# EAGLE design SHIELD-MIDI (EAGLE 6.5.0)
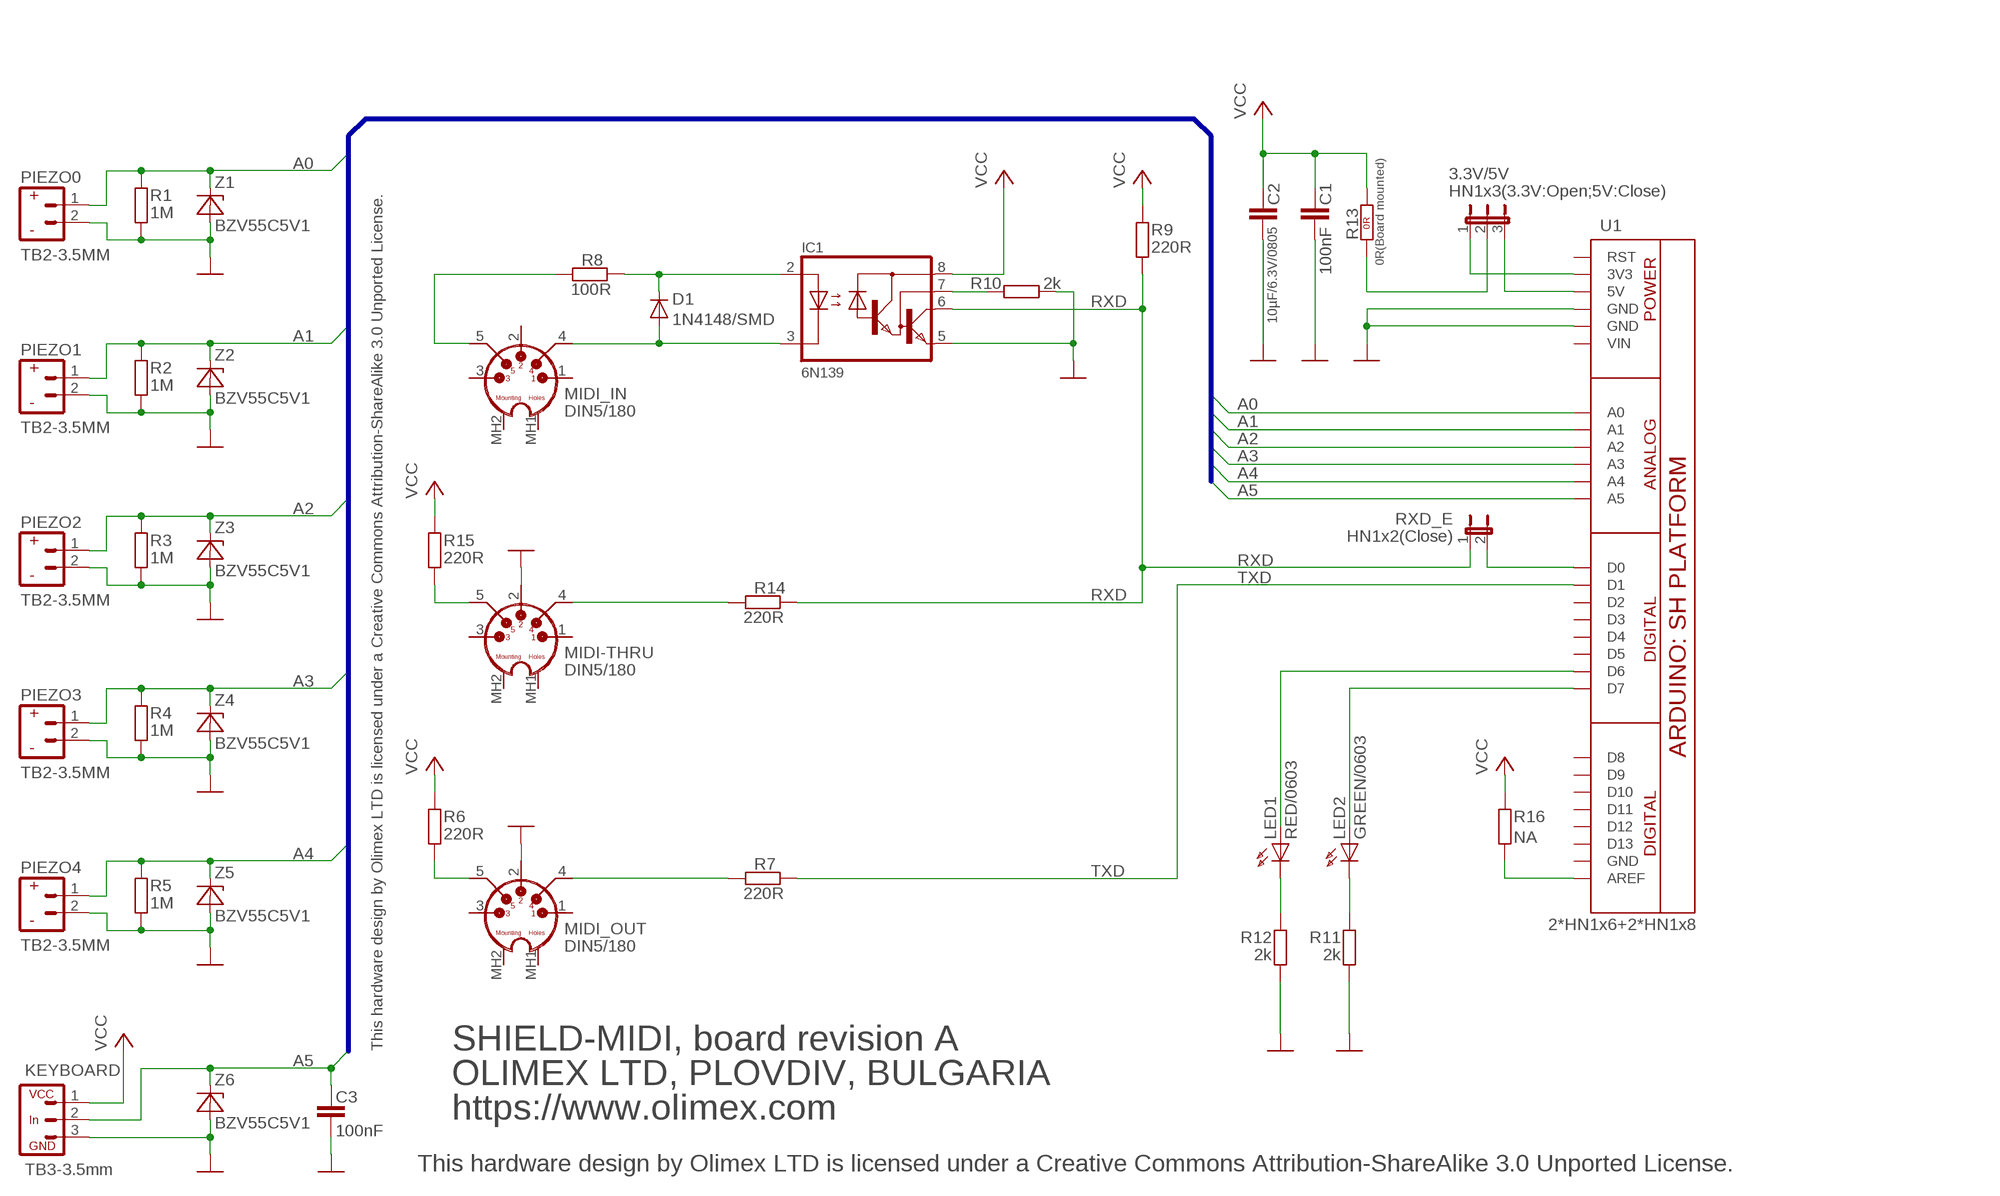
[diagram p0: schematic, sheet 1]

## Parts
3.3V/5V  HN1x3(3.3V:Open;5V:Close)  JP2E  [JP2]
C1  100nF  C-EUC0603_DWS  [C0603_DWS]
C2  10µF/6.3V/0805  C-EUC0805_5MIL_DWS  [C0805_5MIL_DWS]
C3  100nF  C-EUC0603_DWS  [C0603_DWS]
D1  1N4148/SMD  DSMD  [MINI-MELF]
IC1  6N139  HCPL0700  [DIL-08]
KEYBOARD  TB3-3.5mm  CON33.5MM  [CON3/3.5MM]
LED1  RED/0603  LED0603DWS  [LED-0603]
LED2  GREEN/0603  LED0603DWS  [LED-0603]
MIDI-THRU  DIN5/180  MIDI_CON-DIN5/180  [DIN5/180]
MIDI_IN  DIN5/180  MIDI_CON-DIN5/180  [DIN5/180]
MIDI_OUT  DIN5/180  MIDI_CON-DIN5/180  [DIN5/180]
PIEZO0  TB2-3.5MM  CON23.5MM  [CON2/3.5MM]
PIEZO1  TB2-3.5MM  CON23.5MM  [CON2/3.5MM]
PIEZO2  TB2-3.5MM  CON23.5MM  [CON2/3.5MM]
PIEZO3  TB2-3.5MM  CON23.5MM  [CON2/3.5MM]
PIEZO4  TB2-3.5MM  CON23.5MM  [CON2/3.5MM]
R1  1M  R-EU_R0603_5MIL_DWS  [R0603_5MIL_DWS]
R2  1M  R-EU_R0603_5MIL_DWS  [R0603_5MIL_DWS]
R3  1M  R-EU_R0603_5MIL_DWS  [R0603_5MIL_DWS]
R4  1M  R-EU_R0603_5MIL_DWS  [R0603_5MIL_DWS]
R5  1M  R-EU_R0603_5MIL_DWS  [R0603_5MIL_DWS]
R6  220R  R-EU_R0603_5MIL_DWS  [R0603_5MIL_DWS]
R7  220R  R-EU_R0603_5MIL_DWS  [R0603_5MIL_DWS]
R8  100R  R-EU_R0603_5MIL_DWS  [R0603_5MIL_DWS]
R9  220R  R-EU_R0603_5MIL_DWS  [R0603_5MIL_DWS]
R10  2k  R-EU_R0603_5MIL_DWS  [R0603_5MIL_DWS]
R11  2k  R-EU_R0603_5MIL_DWS  [R0603_5MIL_DWS]
R12  2k  R-EU_R0603_5MIL_DWS  [R0603_5MIL_DWS]
R13  0R(Board mounted)  R_0R(NA)  [0805_0R]
R14  220R  R-EU_R0603_5MIL_DWS  [R0603_5MIL_DWS]
R15  220R  R-EU_R0603_5MIL_DWS  [R0603_5MIL_DWS]
R16  NA  R-EU_R0603_5MIL_DWS_NA  [R0603_5MIL_DWS_NA]
RXD_E  HN1x2(Close)  JP1E  [JP1]
U1  2*HN1x6+2*HN1x8  ARDUINO_SH_PLATFORM2  [ARDUINO_MIDI_PLATFORM]
Z1  BZV55C5V1  ZDIOD-SMD  [MINI-MELF]
Z2  BZV55C5V1  ZDIOD-SMD  [MINI-MELF]
Z3  BZV55C5V1  ZDIOD-SMD  [MINI-MELF]
Z4  BZV55C5V1  ZDIOD-SMD  [MINI-MELF]
Z5  BZV55C5V1  ZDIOD-SMD  [MINI-MELF]
Z6  BZV55C5V1  ZDIOD-SMD  [MINI-MELF]

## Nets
3.3V: 3.3V/5V.1 U1.3V3
+5V: 3.3V/5V.3 U1.5V
A0: PIEZO0.1 R1.2 U1.A0 Z1.1(C)
A1: PIEZO1.1 R2.2 U1.A1 Z2.1(C)
A2: PIEZO2.1 R3.2 U1.A2 Z3.1(C)
A3: PIEZO3.1 R4.2 U1.A3 Z4.1(C)
A4: PIEZO4.1 R5.2 U1.A4 Z5.1(C)
A5: C3.1 KEYBOARD.2 U1.A5 Z6.1(C)
GND: C1.2 C2.2 C3.2 IC1.5(GND) KEYBOARD.3 MIDI-THRU.2 MIDI_OUT.2 PIEZO0.2 PIEZO1.2 PIEZO2.2 PIEZO3.2 PIEZO4.2 R1.1 R2.1 R3.1 R4.1 R5.1 R10.1 R11.1 R12.1 U1.GND U1.GND@1(GND) Z1.2(A) Z2.2(A) Z3.2(A) Z4.2(A) Z5.2(A) Z6.2(A)
N$1: R16.1 U1.AREF
N$2: MIDI-THRU.4 R14.2
N$3: 3.3V/5V.2 R13.2(1.2)
N$4: MIDI_OUT.5 R6.1
N$5: RXD_E.2 U1.D0
N$7: MIDI_IN.5 R8.2
N$8: D1.A IC1.3(K) MIDI_IN.4
N$9: D1.C(K) IC1.2(A) R8.1
N$10: LED2.C R11.2
N$11: MIDI-THRU.5 R15.1
N$14: MIDI_OUT.4 R7.2
N$15: LED1.C R12.2
N$23: LED1.A U1.D6
N$24: LED2.A U1.D7
N$53: IC1.7(VB) R10.2
RXD: IC1.6(VO) R9.1 R14.1 RXD_E.1
TXD: R7.1 U1.D1
VCC: C1.1 C2.1 IC1.8(VCC) KEYBOARD.1 R6.2 R9.2 R13.1(1.1) R15.2 R16.2
Unconnected: MIDI-THRU.1 MIDI-THRU.3 MIDI-THRU.MH1 MIDI-THRU.MH2 MIDI_IN.1 MIDI_IN.2 MIDI_IN.3 MIDI_IN.MH1 MIDI_IN.MH2 MIDI_OUT.1 MIDI_OUT.3 MIDI_OUT.MH1 MIDI_OUT.MH2 U1.D2 U1.D3 U1.D4 U1.D5 U1.D8 U1.D9 U1.D10 U1.D11 U1.D12 U1.D13 U1.GND@2(GND) U1.RST U1.VIN

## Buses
A[0..5]

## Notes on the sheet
- +
- -
- +
- -
- +
- -
- +
- -
- +
- -
- This hardware design by Olimex LTD is licensed under a Creative Commons Attribution-ShareAlike 3.0 Unported License. | SHIELD-MIDI, board revision A
- OLIMEX LTD, PLOVDIV, BULGARIA
- VCC
- https://www.olimex.com
- In
- GND
- This hardware design by Olimex LTD is licensed under a Creative Commons Attribution-ShareAlike 3.0 Unported License.

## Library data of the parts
3.3V/5V = jumper:JP2E: JUMPER
C1-C3 = rcl:C-EU: CAPACITOR, European symbol
D1 = DOUBLE-SIDE:D: DIODES
IC1 = OPTOCPL:HCPL0700
KEYBOARD = DOUBLE-SIDE:CON3: CONNECTORS - 3 PINS
LED1 LED2 = DOUBLE-SIDE:LED
MIDI-THRU MIDI_IN MIDI_OUT = OLIMEX_CONNECTORS:MIDI_CON
PIEZO0 PIEZO1-PIEZO4 = DOUBLE-SIDE:CON2: CONNECTORS - 2 PINS
R1-R12 R14-R16 = rcl:R-EU_: RESISTOR, European symbol
R13 = OLIMEX_DISCRET:R_0R
RXD_E = jumper:JP1E: JUMPER
U1 = OLIMEX_CASES:ARDUINO_SH_PLATFORM
Z1-Z6 = gogo:ZDIOD-SMD

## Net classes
1 pwr: width 0.4 mm, drill 0.6 mm, clearance 0.23 mm

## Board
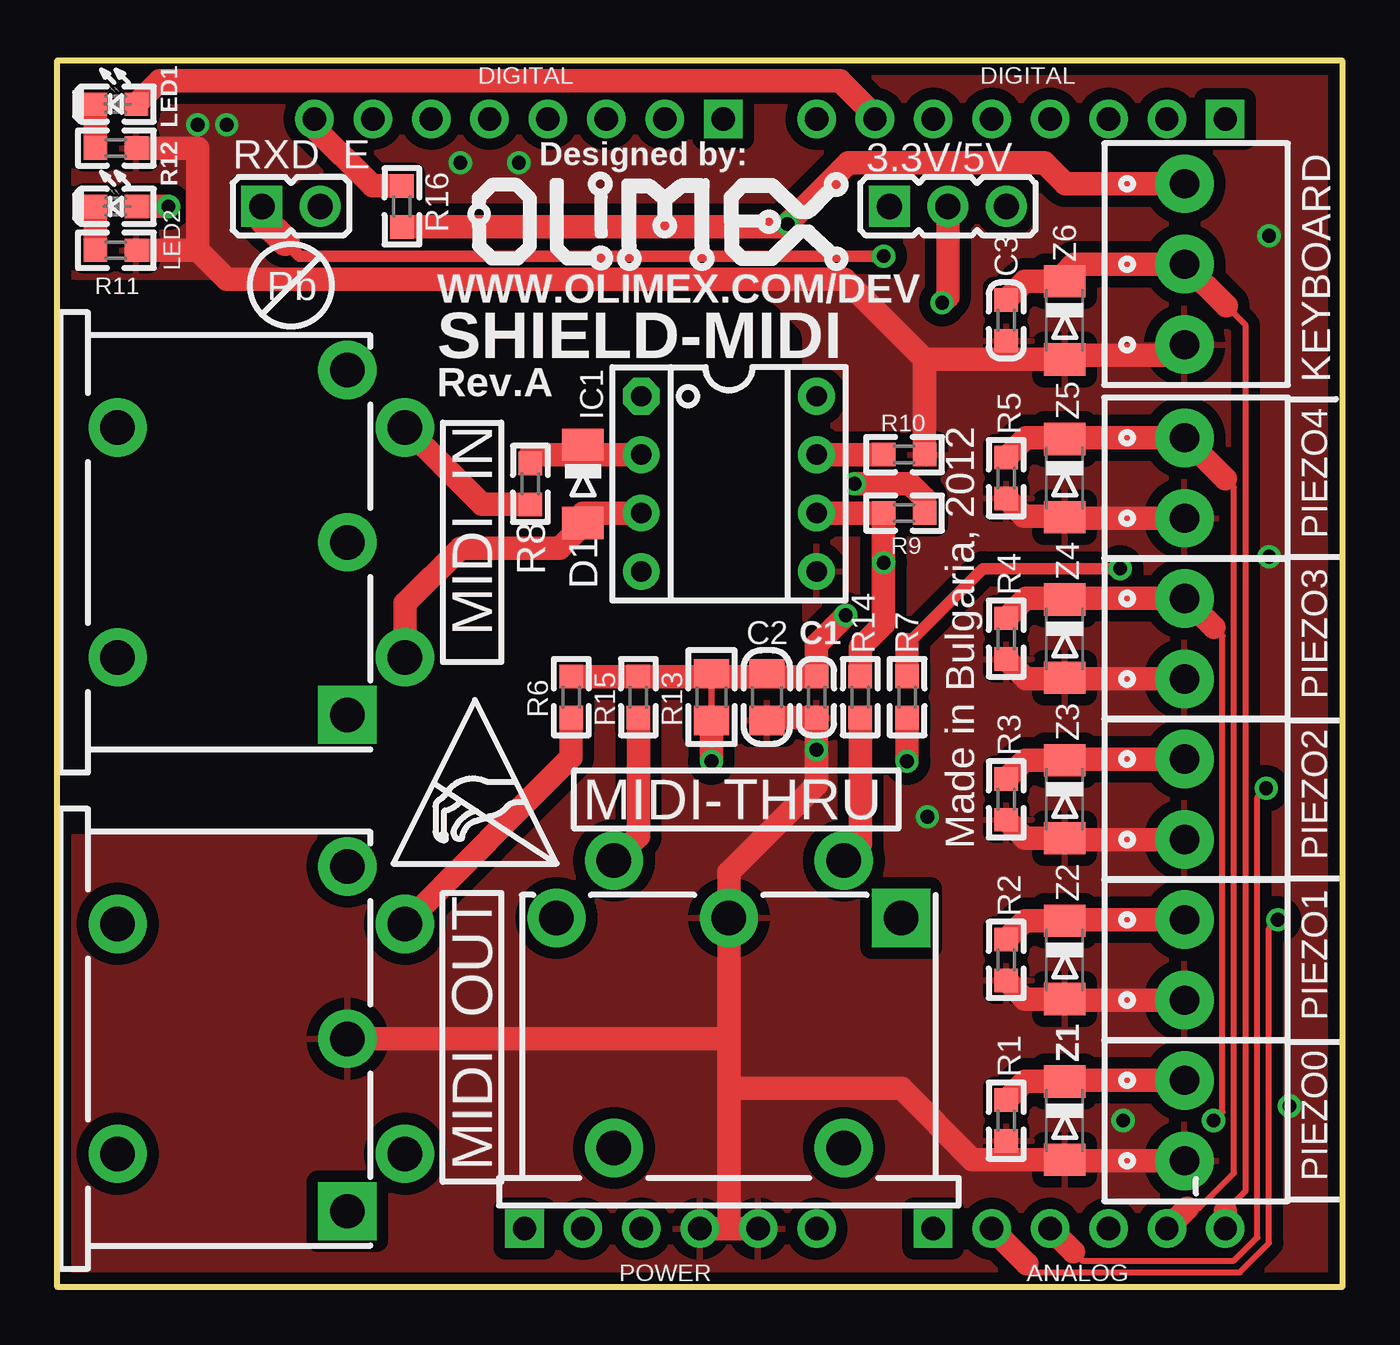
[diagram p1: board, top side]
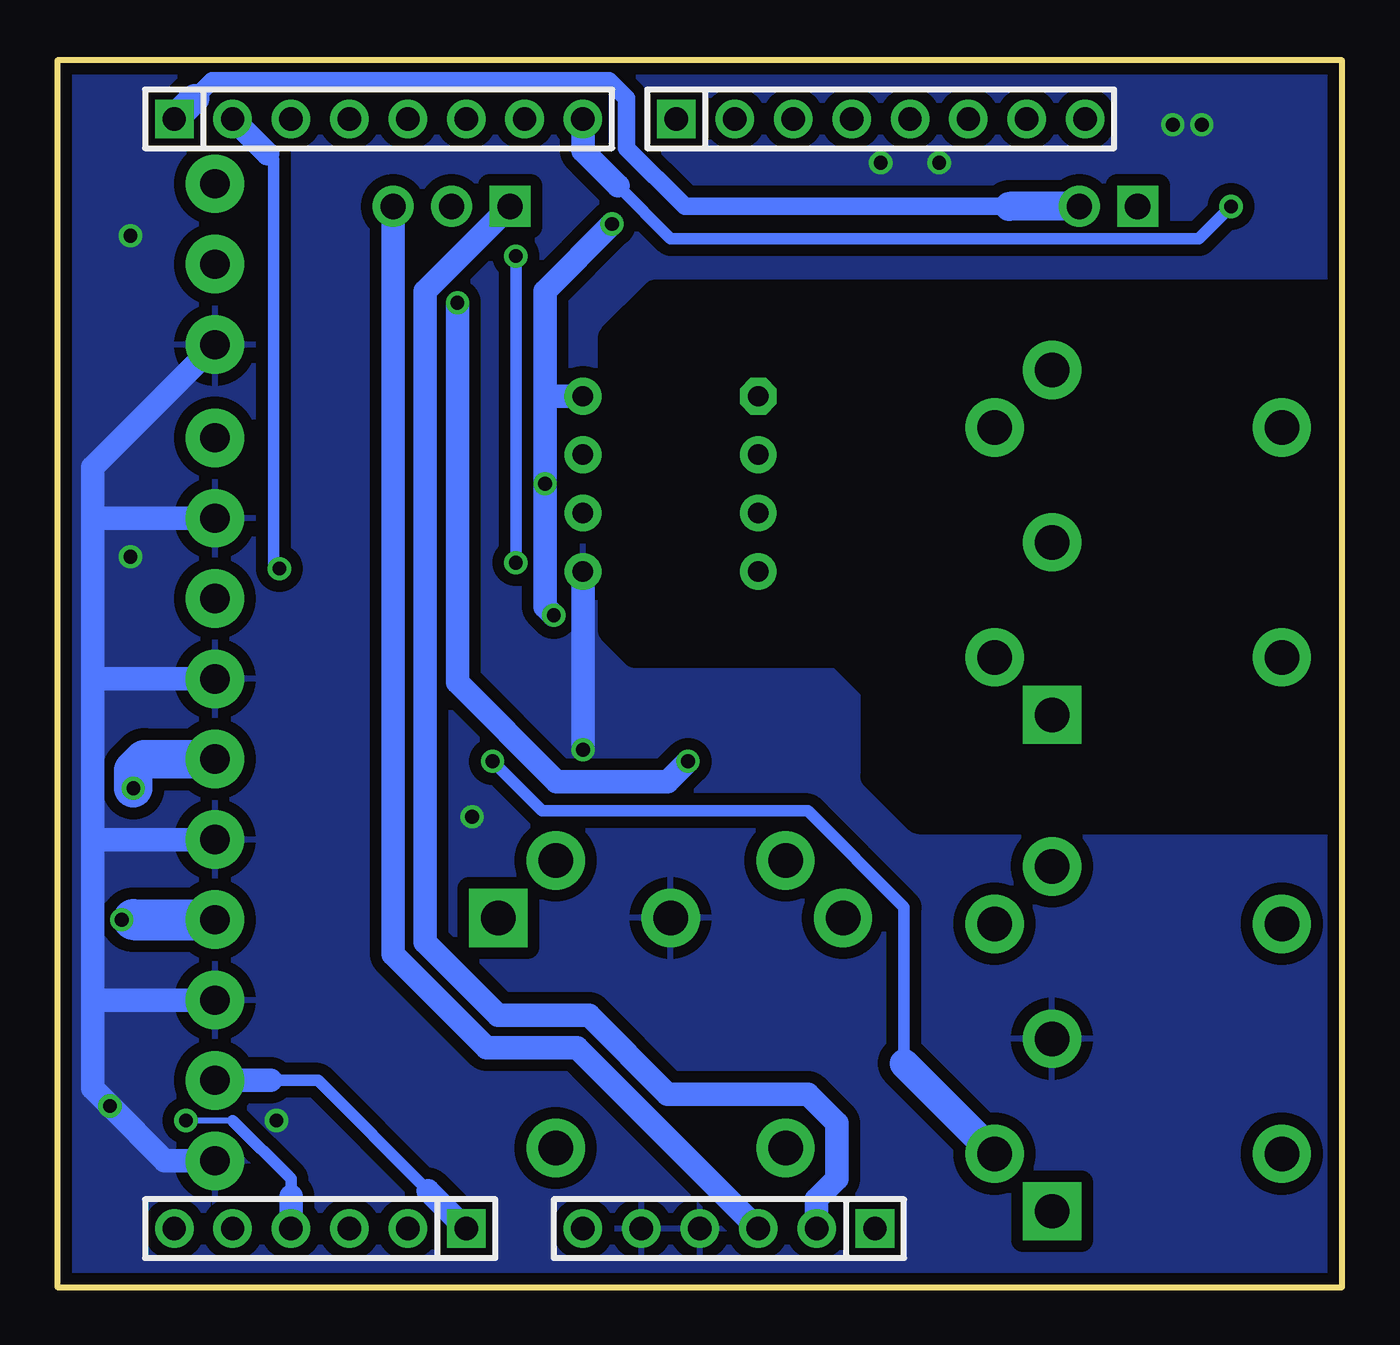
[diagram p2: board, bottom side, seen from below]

Size 55.88 x 53.34 mm. Coordinates in mm from the lower left corner, seen from the top.
Copper layers (1+16): Top 0.035mm / dielectric 1.5mm / Bottom 0.035mm
Design rules "default": minimum track width 10mil, minimum drill 0.6mm, track to track 9.5mil, track to pad 9.5mil, pad to pad 9.5mil, via to via 10mil, smd to smd 1mil, copper to edge 10mil, drill to drill 10mil, minimum pad ring 10mil, minimum via ring 8mil, stop-mask expansion 4mil, vias tented up to drill 25mil, thermal gap 20mil
tRestrict: 9 lines
bRestrict: 9 lines

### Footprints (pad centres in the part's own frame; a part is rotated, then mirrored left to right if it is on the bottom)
JP2 = drill 1.1 pad 1.778 square: 1 -2.54,0 | drill 1.1 pad 1.778: 2 0,0; 3 2.54,0
C0603_DWS = smd 1.016 x 1.016: 1 -0.889,0; 2 0.889,0
C0805_5MIL_DWS = smd 1.27 x 1.524: 1 -1.016,0; 2 1.016,0
MINI-MELF = smd 1.4 x 1.8: A 1.7,0; C -1.7,0
DIL-08 = drill 0.889 pad 1.6 octagon: 1 -3.81,-3.81 | drill 0.889 pad 1.6: 2 -1.27,-3.81; 3 1.27,-3.81; 4 3.81,-3.81; 5 3.81,3.81; 6 1.27,3.81; 7 -1.27,3.81; 8 -3.81,3.81
CON3/3.5MM = drill 1.27 pad 2.54: 1 -1.75,-0.5; 2 1.75,-0.5; 3 5.25,-0.5
LED-0603 = smd 1.016 x 1.016: A 0.889,0; C -0.889,0
DIN5/180 = drill 1.5 pad 2.54 square: 1 7.5,5 | drill 1.5 pad 2.54: 2 0,5; 3 -7.5,5; 4 5,7.5; 5 -5,7.5; MH1 5,-5; MH2 -5,-5
CON2/3.5MM = drill 1.27 pad 2.54: 1 -1.75,-0.5; 2 1.75,-0.5
R0603_5MIL_DWS = smd 1.016 x 1.016: 1 -0.889,0; 2 0.889,0
0805_0R = smd 1.27 x 1.524: 1 -1.016,0; 2 1.016,0
R0603_5MIL_DWS_NA = smd 1.016 x 1.016: 1 -0.889,0; 2 0.889,0
JP1 = drill 1.1 pad 1.778 square: 1 0,-1.27 | drill 1.1 pad 1.778: 2 0,1.27
ARDUINO_MIDI_PLATFORM = drill 1.016 pad 1.676: 3V3 22.86,2.54; 5V 25.4,2.54; A1 40.64,2.54; A2 43.18,2.54; A3 45.72,2.54; A4 48.26,2.54; A5 50.8,2.54; AREF 11.176,50.8; D1 48.26,50.8; D2 45.72,50.8; D3 43.18,50.8; D4 40.64,50.8; D5 38.1,50.8; D6 35.56,50.8; D7 33.02,50.8; D9 26.416,50.8; D10 23.876,50.8; D11 21.336,50.8; D12 18.796,50.8; D13 16.256,50.8; GND 27.94,2.54; GND@1 30.48,2.54; GND@2 13.716,50.8; VIN 33.02,2.54 | drill 1.016 pad 1.676 square: A0 38.1,2.54; D0 50.8,50.8; D8 28.956,50.8; RST 20.32,2.54
MINI-MELF' = smd 1.4 x 1.8: 1 -1.7,0; 2 1.7,0

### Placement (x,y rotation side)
3.3V/5V  38.73,46.99 0 top
C1  33.02,25.65 270 top
C2  30.86,25.65 270 top
C3  41.27,42.04 270 top
D1  22.86,34.92 270 top
IC1  29.21,34.92 270 top
KEYBOARD  49.53,46.23 270 top
LED1  2.54,51.44 0 top
LED2  2.54,46.99 0 top
MIDI-THRU  29.21,11.05 0 top
MIDI_IN  7.62,32.38 270 top
MIDI_OUT  7.62,10.79 270 top
PIEZO0  49.53,7.24 270 top
PIEZO1  49.53,14.22 270 top
PIEZO2  49.53,21.21 270 top
PIEZO3  49.53,28.19 270 top
PIEZO4  49.53,35.18 270 top
R1  41.27,7.24 90 top
R2  41.27,14.22 90 top
R3  41.27,21.21 90 top
R4  41.27,28.19 90 top
R5  41.27,35.18 90 top
R6  22.35,25.65 90 top
R7  36.96,25.65 270 top
R8  20.57,34.92 270 top
R9  36.83,33.66 0 top
R10  36.83,36.2 180 top
R11  2.54,45.09 180 top
R12  2.54,49.53 180 top
R13  28.45,25.65 270 top
R14  34.92,25.65 270 top
R15  25.27,25.65 90 top
R16  14.99,46.99 270 top
RXD_E  10.16,46.99 270 top
U1  0,0 0 top
U$2  [OLIMEX1_V]  35.56,44.07 0 top
U$6  [ESD_SYMBOL]  14.61,18.41 0 top
U$7  [PB_SMALL]  10.16,43.56 0 top
U$8  [RECYCLE_BIN1/8_TOPSTOP]  27.81,9.65 0 bottom
U$9  [LOGO-OPENHARDWARE_8X8_TOPSTOP]  7.62,12.7 0 bottom
Z1  BZV55C5V1  [MINI-MELF']  43.81,7.24 270 top
Z2  BZV55C5V1  [MINI-MELF']  43.81,14.22 270 top
Z3  BZV55C5V1  [MINI-MELF']  43.81,21.21 270 top
Z4  BZV55C5V1  [MINI-MELF']  43.81,28.19 270 top
Z5  BZV55C5V1  [MINI-MELF']  43.81,35.18 270 top
Z6  BZV55C5V1  [MINI-MELF']  43.81,42.04 270 top

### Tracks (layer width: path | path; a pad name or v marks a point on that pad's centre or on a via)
3.3V
  Bottom 1.016: U1.3V3 22.86,3.81 21.97,4.7 21.97,7.11 23.24,8.38 29.34,8.38 32.77,11.81 36.7,11.81 39.88,14.99 39.88,43.31 3.3V/5V.1
+5V
  Bottom 1.016: U1.5V 33.27,10.41 37.21,10.41 41.27,14.48 3.3V/5V.3
A0
  Top 1.016: PIEZO0.1 43.81,8.99 Z1.1 42.09,8.94 R1.2
  Bottom 0.508: 46.61,8.99 44.55,8.99 39.75,4.19
  Bottom 1.016: U1.A0 39.75,4.19 | 46.61,8.99 PIEZO0.1
A1  (via drill 0.6)
  Top 0.254: 42.16,1.02 42.55,0.64 51.44,0.64 52.7,1.91 52.7,15.59 v53.09,15.97
  Top 1.016: PIEZO1.1 43.81,15.97 Z2.1 42.09,15.92 R2.2 | 42.16,1.02 U1.A1
  Bottom 1.016: v53.09,15.97 52.58,15.97
  Bottom 1.778: 52.58,15.97 PIEZO1.1
A2  (via drill 0.6)
  Top 0.254: 44.2,1.52 44.58,1.14 51.18,1.14 52.2,2.16 52.2,21.31 v52.58,21.69
  Top 1.016: PIEZO2.1 43.81,22.96 Z3.1 42.09,22.91 R3.2 | 44.2,1.52 U1.A2
  Bottom 1.676: v52.58,21.69 52.58,22.48 52.1,22.96 PIEZO2.1
A3  (via drill 0.6)
  Top 0.254: 50.29,28.68 50.67,28.3 50.67,7.62 v50.29,7.24
  Top 1.016: 43.81,29.94 PIEZO3.1 50.29,28.68 | 43.81,29.94 Z4.1 | 43.81,29.94 42.14,29.94 R4.2
  Bottom 0.254: 48.26,7.24 v50.29,7.24
  Bottom 0.508: 45.72,3.94 45.72,4.7 48.26,7.24
  Bottom 1.016: U1.A3 45.72,3.94
A4
  Top 0.254: 50.8,35.16 51.18,34.78 51.18,4.95 49.66,3.43 49.15,3.43
  Top 1.016: 43.81,36.93 PIEZO4.1 50.8,35.16 | 43.81,36.93 43.81,36.96 | 43.81,36.93 Z5.1 | 43.81,36.93 42.14,36.93 R5.2 | U1.A4 49.15,3.43
A5
  Top 0.254: 50.84,42.67 51.69,41.82 51.69,4.19 50.8,3.3
  Top 1.016: C3.1 42.09,43.74 Z6.1 43.81,44.07 44.22,44.48 KEYBOARD.2 50.84,42.67 | U1.A5 50.8,3.3
GND  (via drill 0.6)
  Top 1.016: 29.21,8.64 36.7,8.64 39.8,5.54 41.27,5.54 | 41.27,40.34 Z6.2 43.81,40.51 48.56,40.51 KEYBOARD.3 | 41.27,40.34 C3.2 | 41.27,5.54 Z1.2 | 41.27,5.54 R1.1 | C2.2 30.86,24.77 C1.2 v33.02,23.37 33.02,21.84 29.21,18.03 MIDI-THRU.2 29.21,10.79 | R2.1 42.09,12.52 Z2.2 43.81,12.47 PIEZO1.2 | R3.1 42.09,19.51 Z3.2 43.81,19.46 PIEZO2.2 | 43.81,26.44 42.14,26.44 R4.1 | R5.1 42.04,33.53 43.81,33.53 Z5.2 43.81,33.43 PIEZO4.2 | PIEZO3.2 43.81,26.44 | 43.81,26.44 Z4.2 | R12.1 6.1,49.53 6.1,45.09 | 6.1,45.09 R11.1 | 29.21,10.79 29.21,8.64 | 29.21,8.64 29.21,2.54 | 29.21,2.54 U1.GND@1 | 29.21,2.54 U1.GND | MIDI_OUT.2 29.21,10.79 | Z1.2 43.81,5.56 | PIEZO0.2 43.81,5.49 Z1.2 | 41.27,40.34 37.72,40.34 | 37.72,40.34 R10.1 | 37.72,40.34 34.24,43.81 7.37,43.81 6.1,45.09
  Bottom 1.016: PIEZO0.2 51.21,5.49 v53.59,7.87 54.36,8.64 54.36,12.47 | KEYBOARD.3 54.36,35.65 54.36,33.43 | 54.36,12.47 PIEZO1.2 | 54.36,26.44 PIEZO3.2 | 54.36,19.46 54.36,26.44 | 54.36,19.46 PIEZO2.2 | 54.36,12.47 54.36,19.46 | 54.36,33.43 PIEZO4.2 | 54.36,26.44 54.36,33.43 | v33.02,23.37 IC1.5
  other vias: 52.7,31.75 52.7,45.72 46.35,7.24 37.85,20.45 7.37,50.55 20.07,48.9 17.53,48.9 6.1,50.55
  pour Top (isolate 0.508): -2.54,55.88 58.42,55.88 58.42,-2.54 -2.54,-2.54
  pour Bottom (isolate 0.508): -5.08,58.42 60.96,58.42 60.96,-5.08 -5.08,-5.08
N$1
  Top 1.016: R16.1 13.72,47.88 11.18,50.42 U1.AREF
N$2
  Top 1.016: MIDI-THRU.4 34.92,19.26 R14.2
N$3  (via drill 0.6)
  Top 1.016: v28.45,22.86 R13.2 | v38.48,42.8 38.73,43.05 3.3V/5V.2
  Bottom 1.016: v28.45,22.86 29.34,21.97 34.16,21.97 38.48,26.29 v38.48,42.8
N$4
  Top 1.016: MIDI_OUT.5 22.35,23.03 R6.1
N$5
  Bottom 0.762: 49.91,51.69 49.15,52.45 31.88,52.45 31.11,51.69 31.11,49.53 28.57,46.99 14.48,46.99
  Bottom 1.27: 49.91,51.69 U1.D0 | RXD_E.2 14.48,46.99
N$7
  Top 1.016: MIDI_IN.5 18.47,34.04 R8.2
N$8
  Top 1.016: IC1.3 22.86,33.66 D1.A 22.86,33.15 21.84,32.13 17.53,32.13 15.12,29.73 MIDI_IN.4
N$9
  Top 1.016: 22.86,36.2 D1.C | 22.86,36.2 IC1.2 | R8.1 20.57,36.2 22.86,36.2
N$10
  Top 1.016: R11.2 LED2.C
N$11
  Top 1.016: MIDI-THRU.5 25.27,19.61 R15.1
N$14  (via drill 0.6)
  Top 1.016: v36.96,22.86 R7.2
  Bottom 0.508: 19.05,9.72 19.05,16.51 23.24,20.7 34.8,20.7 v36.96,22.86
  Bottom 1.27: MIDI_OUT.4 19.05,9.72
N$15
  Top 1.016: R12.2 LED1.C
N$23
  Top 1.016: U1.D6 35.56,50.93 34.04,52.45 4.45,52.45 LED1.A
N$24  (via drill 0.6)
  Top 1.016: LED2.A v4.83,46.99
  Bottom 0.508: v4.83,46.99 6.22,45.59 29.21,45.59 31.5,47.88
  Bottom 1.016: 31.5,47.88 33.02,49.4 U1.D7
N$53
  Top 1.016: IC1.7 R10.2
RXD  (via drill 0.6)
  Top 0.508: 9.91,45.47 10.54,44.83 v35.94,44.83
  Top 1.016: IC1.6 R9.1 v35.94,31.5 35.94,28.83 34.92,27.81 R14.1
  Top 1.27: RXD_E.1 8.89,46.48 9.91,45.47
  Bottom 0.508: v35.94,44.83 v35.94,31.5
TXD  (via drill 0.6)
  Top 0.508: 36.96,27.94 40.26,31.24 v46.23,31.24
  Top 1.016: R7.1 36.96,27.94
  Bottom 0.508: v46.23,31.24 46.48,31.5 46.48,49.02 46.74,49.28
  Bottom 1.016: 46.74,49.28 U1.D1
VCC  (via drill 0.6)
  Top 1.016: R6.2 R15.2 28.45,26.54 | 28.45,26.54 R13.1 | 30.86,26.54 C2.1 | 28.45,26.54 30.86,26.54 | 30.86,26.54 C1.1 33.02,27.94 v34.29,29.21 | R16.2 31.62,46.1 v31.75,46.23 34.42,48.9 42.93,48.9 43.84,47.98 KEYBOARD.1 | R9.2 37.72,34.29 37.08,34.92 v34.67,34.92
  Bottom 1.016: v34.29,29.21 34.67,29.59 v34.67,34.92 34.67,38.73 | 34.67,38.73 34.67,43.31 v31.75,46.23 | 34.67,38.73 IC1.8

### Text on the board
tNames: Designed by: | WWW.OLIMEX.COM/DEV | SHIELD-MIDI | Rev.A | Made in Bulgaria, 2012 | Without bottom silk!!!!
bStop: VCC | IN | GND | + | - | + | - | + | - | + | - | + | - | RoHS | Compliant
